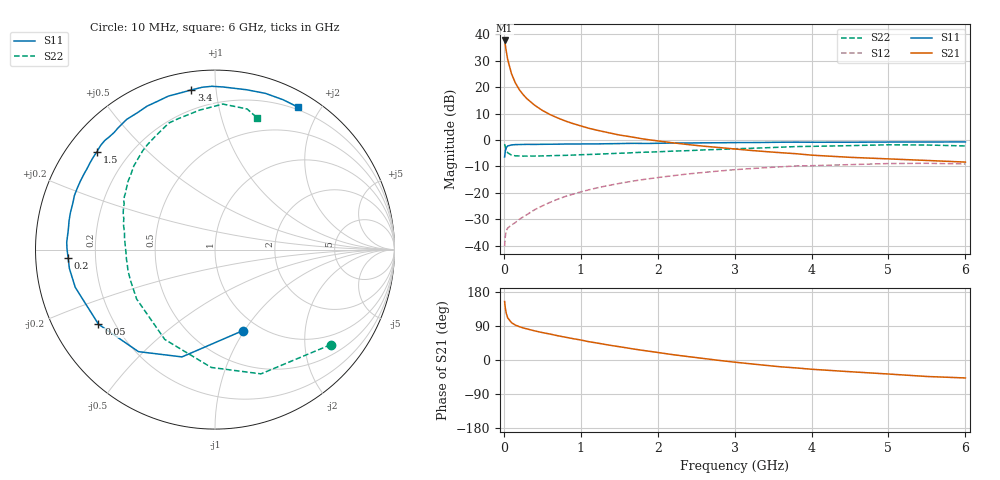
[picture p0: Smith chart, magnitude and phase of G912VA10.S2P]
! SIEMENS Small Signal Semiconductors
! BFG235
! Si NPN RF Bipolar Junction Transistor in SOT223
! VCE = 12 V  IC = 100 mA
! Common Emitter S-Parameters:  July  1994
# GHz  S  MA  R  50
!  f  S11  S21  S12  S22
! GHz  MAG  ANG  MAG  ANG  MAG  ANG  MAG  ANG
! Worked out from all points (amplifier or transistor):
!   40 points, 10 MHz to 6 GHz, reference 50 ohm
!   highest |S21| = 37.7 dB at 10 MHz (marker M1)
!   |S21| within 3 dB of that: start of sweep to 25.9 MHz
!   unconditionally stable (mu >= 1): 489.2 MHz to 1.475 GHz
!   at 200 MHz: K = 0.75, MSG = 24.6 dB, |S12| = -30.1 dB
!   at 1.5 GHz: K = 1.00, MSG = 9.2 dB, |S12| = -16.4 dB
!   at 6 GHz: K = 0.90, MSG = 0.4 dB, |S12| = -9.1 dB
!   S11 on the Smith chart (normalised r, x): 10 MHz: 0.84, -0.99; 50 MHz: 0.14, -0.29; 200 MHz: 0.10, -0.03; 1.5 GHz: 0.09, +0.36; 3.4 GHz: 0.09, +0.86; 6 GHz: 0.17, +1.73
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0.01  0.4773 -70.8  76.41 154.5  0.0098 64.5  0.8344 -39.4
0.02  0.6255 -107.1  61.73 136.2  0.0153 50.1  0.7382 -69.7
0.03  0.7108 -126.9  49.36 124.4  0.0189 42.3  0.657 -91.8
0.05  0.771 -147.4  33.43 111.2  0.0216 33.7  0.5736 -119.2
0.1  0.8065 -164.9  17.83 98.4  0.0246 33.7  0.5162 -147.8
0.15  0.8181 -172.6  12.02 92.1  0.0275 39.6  0.5013 -159.8
0.2  0.8193 -176.7  8.997 88.1  0.0314 43.6  0.499 -166.3
0.25  0.8243 180.0  7.246 84.7  0.0351 47.5  0.4957 -170.6
0.3  0.8271 177.2  6.05 82.1  0.0387 51.1  0.4963 -174.0
0.4  0.8247 172.5  4.55 76.9  0.0479 54.9  0.4964 -178.6
0.5  0.8288 168.7  3.633 72.4  0.0566 57.0  0.5001 177.9
0.6  0.8316 165.5  3.033 68.5  0.066 58.1  0.5043 174.8
0.7  0.8333 161.9  2.611 64.0  0.0758 58.4  0.5092 172.1
0.9  0.8402 156.3  2.043 56.3  0.0944 57.2  0.5185 167.6
1.1  0.8427 150.0  1.674 48.5  0.1137 55.2  0.5324 163.1
1.5  0.8544 140.4  1.244 35.1  0.1507 49.5  0.5611 155.1
2.2  0.8766 124.2  0.883 14.0  0.2114 37.5  0.6161 141.8
3.2  0.8937 102.7  0.637 -9.9  0.2869 18.3  0.6963 122.5
3.4  0.8994 98.4  0.604 -14.0  0.2991 14.1  0.7125 118.0
4.5  0.9079 78.8  0.47 -30.9  0.3419 -7.1  0.7815 96.4
5.5  0.9171 65.6  0.41 -43.5  0.3622 -25.7  0.8036 77.1
6  0.9189 59.7  0.382 -47.4  0.3516 -32.5  0.7708 72.3
